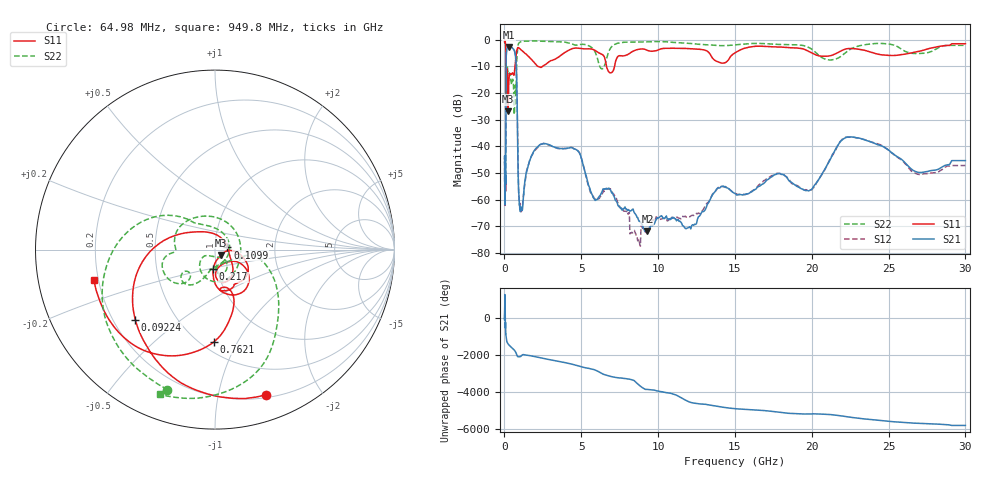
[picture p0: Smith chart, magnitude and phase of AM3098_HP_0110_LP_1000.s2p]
! Date/Time: Thu, Feb 28, 2019 8:37 AM
! Network Analyzer: Agilent Technologies E8364B Rev: A.07.50.67
! Sweep from 0.010 to 30.000 GHz, 1601 Points, Sweep Type: LOG
! Power Supply: 5.023 V, 0.002 A
# Hz S DB R 50
!freq MagS11 AngS11 MagS21 AngS21 MagS12 AngS12 MagS22 AngS22
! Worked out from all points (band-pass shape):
!   1601 points, 10 MHz to 30 GHz, reference 50 ohm
!   highest |S21| = -2.76 dB at 293 MHz (marker M1); lowest = -71.8 dB at 9.302 GHz (marker M2)
!   |S21| within 3 dB of the highest: 118.1 MHz to 706.4 MHz (588.3 MHz wide, 143 % of centre)
!   lowest |S11| = -26.9 dB at 239.9 MHz (marker M3), VSWR 1.09, Z = 53.4 - j3.21 ohm
!   |S11| at or under -10 dB: 99.91 MHz to 682.8 MHz (582.9 MHz wide, 149 % of centre); 2.163 GHz to 2.513 GHz (349.6 MHz wide, 15 % of centre); 6.641 GHz to 7.168 GHz (526.8 MHz wide, 7.63 % of centre)
!   |S22| runs from -28.1 to -0.5 dB; largest |S21 - S12| = 0.011
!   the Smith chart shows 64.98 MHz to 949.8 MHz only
!   S11 on the Smith chart (normalised r, x): 64.98 MHz: 0.23, -1.39; 92.24 MHz: 0.29, -0.35; 109.9 MHz: 1.15, +0.03; 217 MHz: 0.96, -0.21; 762.1 MHz: 0.58, -0.81; 949.8 MHz: 0.18, -0.12
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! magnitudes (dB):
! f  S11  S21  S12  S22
! 10 MHz  -0.4  -44.7  -46.3  -0.6
! 38.04 MHz  -0.5  -59.4  -58.6  -0.9
! 64.98 MHz  -1.3  -53.6  -52.1  -1.7
! 79.38 MHz  -2.1  -52.3  -54.1  -2.5
! 92.24 MHz  -4.6  -34.5  -34.6  -5.0
! 109.9 MHz  -23.1  -7.9  -7.9  -17.7
! 144.7 MHz  -19.1  -3.8  -3.7  -14.1
! 217 MHz  -19.1  -3.0  -3.0  -11.8
! 239.9 MHz  -26.9  -2.9  -2.8  -12.7
! 293 MHz  -15.1  -2.8  -2.7  -12.8
! 550.5 MHz  -12.7  -3.4  -3.4  -15.0
! 639.6 MHz  -12.7  -4.1  -4.0  -28.1
! 762.1 MHz  -5.8  -9.5  -9.4  -18.1
! 949.8 MHz  -3.2  -58.8  -60.3  -1.3
! 1.149 GHz  -4.2  -63.5  -63.2  -0.7
! 2.084 GHz  -9.6  -40.6  -41.0  -0.6
! 4.663 GHz  -3.2  -41.2  -41.2  -2.1
! 7.926 GHz  -5.9  -63.4  -64.4  -1.0
! 9.302 GHz  -4.1  -71.8  -71.9  -0.9
! 19.7 GHz  -4.2  -56.5  -56.3  -2.7
! 22.67 GHz  -3.4  -36.5  -36.6  -3.2
! 30 GHz  -1.6  -45.3  -47.2  -2.2
